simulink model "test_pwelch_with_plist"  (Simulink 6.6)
settings: Solver=ode45  StartTime=0.0  StopTime=10.0  RelTol=1e-3
libraries: sltpda x5

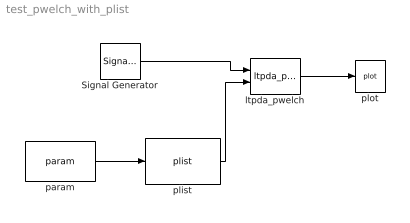
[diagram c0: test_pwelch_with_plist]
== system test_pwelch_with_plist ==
  Signal Generator : sltpda/AO class/Signal Generator  Tag=ao  SystemSampleTime=-1  nsecs=10  fs=100  tsfcn=sin(2*pi*10*t)
  ltpda_pwelch : sltpda/Signal Processing blocks/Frequency domain/ltpda_pwelch  Tag=ltpda_pwelch  Description=Makes a spectral density estimate by calling ltpda_pwlech.  SystemSampleTime=-1  win=Hanning  nfft=0  psll=0  nolap=0
  param : sltpda/AO class/param  SystemSampleTime=-1  key=Nfft  value=100
  plist : sltpda/AO class/plist  SystemSampleTime=-1
  plot : sltpda/AO class/plot  Tag=plot  Description=Plot an analysis object.  SystemSampleTime=-1  xscale=linear  yscale=linear
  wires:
  Signal Generator/1 -> ltpda_pwelch/1
  ltpda_pwelch/1 -> plot/1
  plist/1 -> ltpda_pwelch/2
  param/1 -> plist/1
